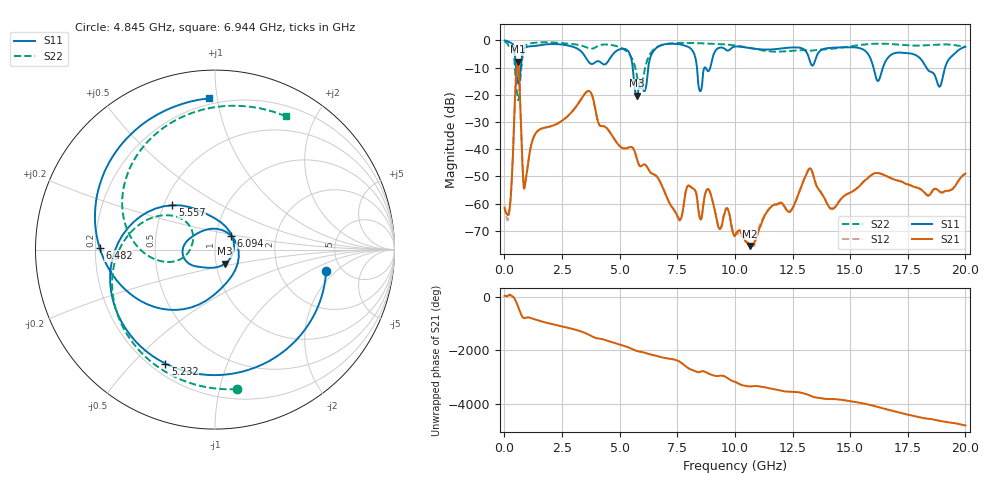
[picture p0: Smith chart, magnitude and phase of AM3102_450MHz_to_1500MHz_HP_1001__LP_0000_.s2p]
!Agilent Technologies,E8364B,MY43040894,A.07.50.67
!Agilent E8364B: A.07.50.67
!Date: Thursday, January 11, 2018 06:00:51
!Correction: S11(Full 2 Port(1,2))
!S21(Full 2 Port(1,2))
!S12(Full 2 Port(1,2))
!S22(Full 2 Port(1,2))
!S2P File: Measurements: S11, S21, S12, S22:
# Hz S  dB  R 50
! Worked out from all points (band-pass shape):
!   1601 points, 10 MHz to 20 GHz, reference 50 ohm
!   highest |S21| = -7.84 dB at 584.7 MHz (marker M1); lowest = -75.5 dB at 10.64 GHz (marker M2)
!   |S21| within 3 dB of the highest: 530 MHz to 629.2 MHz (99.14 MHz wide, 17.1 % of centre)
!   lowest |S11| = -20.3 dB at 5.745 GHz (marker M3), VSWR 1.21, Z = 55.3 - j8.69 ohm
!   |S11| at or under -10 dB: 5.568 GHz to 6.243 GHz (675.7 MHz wide, 11.4 % of centre); 16.01 GHz to 16.42 GHz (411.1 MHz wide, 2.54 % of centre); 18.3 GHz to 19.12 GHz (816.7 MHz wide, 4.36 % of centre)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
!   |S22| runs from -22.0 to -0.4 dB; largest |S21 - S12| = 0.0015
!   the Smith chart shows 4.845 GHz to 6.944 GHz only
!   S11 on the Smith chart (normalised r, x): 4.845 GHz: 3.77, -1.50; 5.232 GHz: 0.26, -0.62; 5.557 GHz: 0.55, +0.31; 6.094 GHz: 1.18, +0.19; 6.482 GHz: 0.22, +0.01; 6.944 GHz: 0.16, +0.95
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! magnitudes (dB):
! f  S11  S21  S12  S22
! 10 MHz  -0.1  -61.7  -60.9  -0.4
! 234.9 MHz  -0.7  -61.4  -61.4  -2.7
! 584.7 MHz  -15.5  -7.8  -7.9  -21.4
! 897.1 MHz  -2.8  -52.7  -52.7  -2.1
! 1.372 GHz  -2.0  -34.0  -34.0  -0.9
! 3.346 GHz  -4.2  -21.4  -21.4  -2.0
! 4.845 GHz  -4.0  -37.3  -37.3  -2.1
! 5.232 GHz  -3.2  -39.8  -39.8  -3.6
! 5.557 GHz  -9.3  -39.4  -39.4  -7.1
! 5.745 GHz  -20.3  -43.4  -43.5  -12.6
! 6.094 GHz  -18.5  -45.6  -45.7  -10.5
! 6.482 GHz  -3.8  -49.3  -49.2  -3.4
! 6.682 GHz  -2.3  -50.8  -50.8  -2.2
! 6.944 GHz  -1.5  -55.5  -55.7  -1.5
! 8.493 GHz  -18.7  -65.6  -65.4  -1.1
! 10.01 GHz  -2.3  -71.8  -71.5  -1.9
! 10.64 GHz  -2.8  -75.5  -75.2  -2.8
! 13.34 GHz  -9.2  -48.0  -47.9  -3.8
! 14.2 GHz  -2.7  -62.0  -61.7  -3.1
! 16.68 GHz  -6.1  -50.3  -50.3  -1.3
! 18.88 GHz  -17.1  -55.6  -55.5  -1.5
! 20 GHz  -2.4  -49.0  -48.9  -2.3
